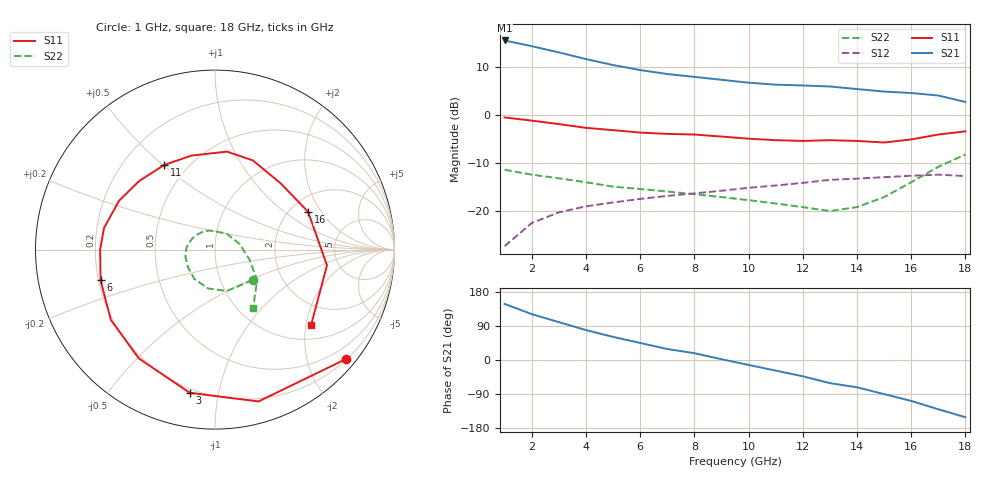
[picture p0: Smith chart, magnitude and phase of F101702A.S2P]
!ATF-10170
!S-PARAMETERS at Vds=2V  Id=25mA.  LAST UPDATED 07-22-92
# ghz s ma r 50
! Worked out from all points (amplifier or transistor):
!   18 points, 1 GHz to 18 GHz, reference 50 ohm
!   highest |S21| = 15.6 dB at 1 GHz (marker M1)
!   |S21| within 3 dB of that: start of sweep to 3.365 GHz
!   unconditionally stable (mu >= 1): 10.08 GHz to end of sweep
!   at 4 GHz: K = 0.57, MSG = 15.4 dB, |S12| = -19.0 dB
!   at 10 GHz: K = 1.00, MSG = 11.0 dB, |S12| = -15.1 dB
!   at 18 GHz: K = 1.12, MAG = 5.6 dB, |S12| = -12.7 dB
!   lowest NFmin = 0.30 dB at 100 MHz
!   S11 on the Smith chart (normalised r, x): 1 GHz: 0.22, -2.73; 3 GHz: 0.18, -0.82; 6 GHz: 0.21, -0.13; 11 GHz: 0.37, +0.50; 16 GHz: 2.49, +1.52; 18 GHz: 1.38, -2.14
1  0.95 -40.0  6.05 148.0  0.043 66.0  0.27 -39.0
2  0.88 -74.0  5.27 121.0  0.075 47.0  0.24 -74.0
3  0.81 -100.0  4.54 100.0  0.097 34.0  0.22 -100.0
4  0.74 -125.0  3.87 79.0  0.112 22.0  0.2 -125.0
5  0.7 -146.0  3.35 61.0  0.123 11.0  0.18 -146.0
6  0.66 -165.0  2.97 45.0  0.134 1.0  0.17 -166.0
7  0.64 180.0  2.7 29.0  0.144 -8.0  0.16 177.0
8  0.63 169.0  2.52 18.0  0.153 -13.0  0.15 166.0
9  0.6 153.0  2.35 2.0  0.163 -23.0  0.14 153.0
10  0.57 138.0  2.19 -13.0  0.175 -34.0  0.13 140.0
11  0.55 121.0  2.09 -28.0  0.185 -44.0  0.12 123.0
12  0.54 104.0  2.05 -43.0  0.197 -56.0  0.11 105.0
13  0.55 83.0  2 -61.0  0.212 -69.0  0.1 82.0
14  0.54 67.0  1.88 -72.0  0.218 -80.0  0.11 54.0
15  0.52 45.0  1.77 -90.0  0.226 -93.0  0.14 13.0
16  0.56 22.0  1.71 -108.0  0.234 -108.0  0.2 -16.0
17  0.63 -8.0  1.61 -130.0  0.24 -126.0  0.29 -36.0
18  0.68 -38.0  1.38 -151.0  0.232 -144.0  0.39 -57.0
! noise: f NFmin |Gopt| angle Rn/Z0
0.1  0.3  0.99  1  0.5
2  0.4  0.73  47  0.34
4  0.5  0.46  95  0.17
6  0.7  0.44  131  0.3
8  0.9  0.43  162  0.44
12  1.3  0.37  -121  0.7
